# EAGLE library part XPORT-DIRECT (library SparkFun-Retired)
TCP/IP phy and stack module
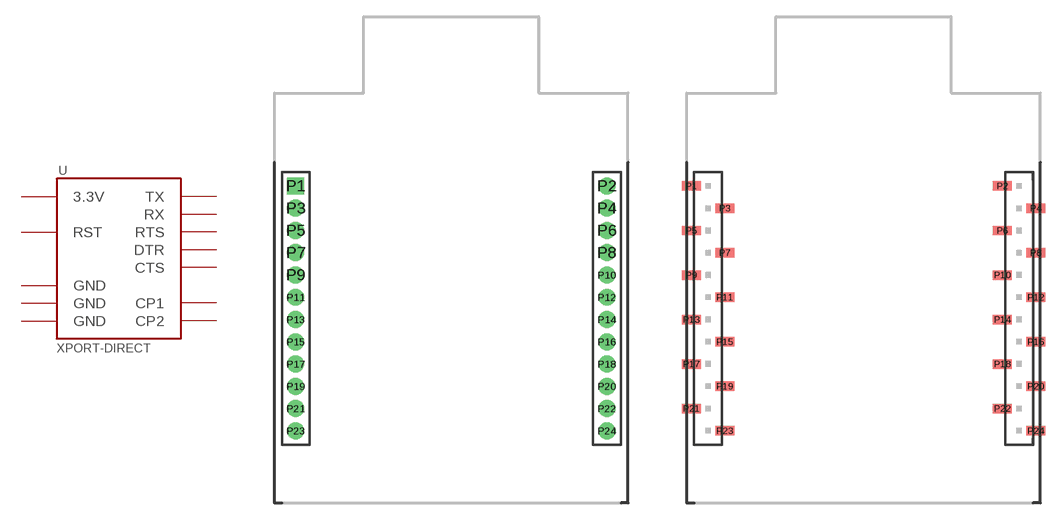
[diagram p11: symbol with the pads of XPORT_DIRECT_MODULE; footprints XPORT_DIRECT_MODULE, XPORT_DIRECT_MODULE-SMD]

Designator prefix -

## XPORT-DIRECT  [XPORT_DIRECT_MODULE]
P1  GND
P2  GND
P3  3.3V
P5  RST
P7  TX
P9  RX
P11  RTS
P13  DTR
P15  CTS
P21  CP2
P23  CP1
P24  GND

## XPORT-DIRECTSMD  [XPORT_DIRECT_MODULE-SMD]
Pads as for XPORT_DIRECT_MODULE

## Footprint XPORT_DIRECT_MODULE (pad centres in mm)
drill 0.8 pad 1.524 square: P1 -13.97,9.3
drill 0.8 pad 1.524: P2 13.97,9.3; P3 -13.97,7.3; P4 13.97,7.3; P5 -13.97,5.3; P6 13.97,5.3; P7 -13.97,3.3; P8 13.97,3.3; P9 -13.97,1.3; P10 13.97,1.3; P11 -13.97,-0.7; P12 13.97,-0.7; P13 -13.97,-2.7; P14 13.97,-2.7; P15 -13.97,-4.7; P16 13.97,-4.7; P17 -13.97,-6.7; P18 13.97,-6.7; P19 -13.97,-8.7; P20 13.97,-8.7; P21 -13.97,-10.7; P22 13.97,-10.7; P23 -13.97,-12.7; P24 13.97,-12.7

## Footprint XPORT_DIRECT_MODULE-SMD (pad centres in mm)
smd 1.7 x 0.85: P1 -15.472,9.294; P2 12.468,9.294; P3 -12.472,7.294; P4 15.468,7.294; P5 -15.472,5.293; P6 12.468,5.293; P7 -12.472,3.294; P8 15.468,3.294; P9 -15.472,1.293; P10 12.468,1.293; P11 -12.472,-0.707; P12 15.468,-0.707; P13 -15.472,-2.707; P14 12.468,-2.707; P15 -12.472,-4.707; P16 15.468,-4.707; P17 -15.472,-6.707; P18 12.468,-6.707; P19 -12.472,-8.707; P20 15.468,-8.707; P21 -15.472,-10.707; P22 12.468,-10.707; P23 -12.472,-12.707; P24 15.468,-12.707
